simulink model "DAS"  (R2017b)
settings: Solver=FixedStepDiscrete  StartTime=0.0  StopTime=10.0  FixedStep=0.01  RelTol=1e-3  EnableMultiTasking=on
undefined symbols (not defined in the file): CcDAS_ACModeCurtLim_A, CcDAS_ACModeCurtTiLim_ms, CcDAS_BMSOperationConfirmTi_ms, CcDAS_CellMaxTempLim1_C, CcDAS_CellMaxTempLim2_C, CcDAS_CellMaxTempLim3_C, CcDAS_CellMaxTempLim4_C, CcDAS_CellMinTempHiLim_C, CcDAS_CellMinTempLowLim_C, CcDAS_CellMinTempMidLim_C, CcDAS_CellTempDiffLim_C, CcDAS_DCModeCurtTiLim_ms, CcDAS_HVSafetyNVMStoreTi_ms, CcDAS_OCVSOCDiffLim1_numb, CcDAS_OCVSOCDiffLim2_numb, CcDAS_PackCurrLim_A, CcDAS_SOCHighLim_numb, CcDAS_SOCLowerLim_numb, CcDAS_SOHLowerLim_numb, CcDAS_SOHLowerLimSale_numb, DAS_MIN2MS_NUMB, DAS_RUNTIME100_MS, DAS_RUNTIME10_MS, DAS_STATSTIMEMAX_MIN, DAS_STATSTIMEMIN_MIN, DAS_STATSTIMESMAX_NUMB, DAS_STATSTIMESMIN_NUMB, DAS_TIMESONE_NUMB, Enum_CTCCtrCtlConnMode
libraries: AIWAYS_Powertrain_BMS_lib x268
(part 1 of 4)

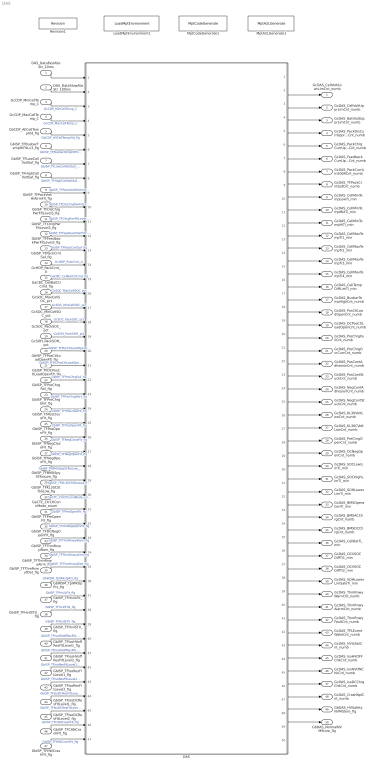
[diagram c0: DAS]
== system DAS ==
  DAS_DataFastAbsStr_10ms : Inport
  DAS_DataSlowAbsStr_100ms : Inport  Port=2
  GcCDP_MinCellTemp_C : Inport  Port=3
  GcCDP_MaxCellTemp_C : Inport  Port=4
  GbCDP_AllCellTempVld_flg : Inport  Port=5
  GbISP_TFBusbarTempHiFltLv3_flg : Inport  Port=6
  GbISP_TFLowCellVoltSaf_flg : Inport  Port=7
  GbISP_TFHighCellVoltSaf_flg : Inport  Port=8
  GbISP_TFPackVoltHiAlrmFlt_flg : Inport  Port=9
  GbISP_TFDisChrgPwrFltLevel3_flg : Inport  Port=10
  GbISP_TFChrgPwrFltLevel3_flg : Inport  Port=11
  GbISP_TFFeedbackPwrFltLevel3_flg : Inport  Port=12
  GbISP_TFPackCrntSaf_flg : Inport  Port=13
  GcHDP_PackCrnt_A : Inport  Port=14
  GaCBC_CellBalCtlCmd_flg : Inport  Port=15
  GcSOC_MaxCellSOC_pct : Inport  Port=16
  GcSOC_MinCellSOC_pct : Inport  Port=17
  GcSOC_PackSOC_pct : Inport  Port=18
  GcSOH_PackSOH_pct : Inport  Port=19
  GbISP_TFPosCtlLoadOpenFlt_flg : Inport  Port=20
  GbISP_TFDCPosCtlLoadOpenFlt_flg : Inport  Port=21
  GbISP_TFPreChrgFail_flg : Inport  Port=22
  GbISP_TFPreChrgShrt_flg : Inport  Port=23
  GbISP_TFPosCloseFlt_flg : Inport  Port=24
  GbISP_TFPosOpenFlt_flg : Inport  Port=25
  GbISP_TFNegCloseFlt_flg : Inport  Port=26
  GbISP_TFNegOpenFlt_flg : Inport  Port=27
  GbISP_TFBMUSpyStTooLow_flg : Inport  Port=28
  GbISP_TFKL30CStTooLow_flg : Inport  Port=29
  GeCTC_CtrCtlConnMode_enum : Inport  Port=30
  GbISP_TFPreOpenFlt_flg : Inport  Port=31
  GbISP_TFDCNegOpenFlt_flg : Inport  Port=32
  GbISP_TFThmRnwyWarn_flg : Inport  Port=33
  GbISP_TFThmRnwyAlrm_flg : Inport  Port=34
  GbISP_TFThmRnwyfDet_flg : Inport  Port=35
  GbWSM_TplWkUpPrs_flg : Inport  Port=36
  GbISP_TFHvilLFlt_flg : Inport  Port=37
  GbISP_TFHvilSTG_flg : Inport  Port=38
  GbISP_TFHvilSTV_flg : Inport  Port=39
  GbISP_TFIsoHVoffResFltLevel1_flg : Inport  Port=40
  GbISP_TFIsoHVoffResFltLevel2_flg : Inport  Port=41
  GbISP_TFIsoResFltLevel1_flg : Inport  Port=42
  GbISP_TFIsoResFltLevel2_flg : Inport  Port=43
  GbISP_TFIsoDCResFltLevel1_flg : Inport  Port=44
  GbISP_TFIsoDCResFltLevel2_flg : Inport  Port=45
  GbISP_TFCANCrashFlt_flg : Inport  Port=46
  GbISP_TFHWCrashFlt_flg : Inport  Port=47
  DAS : Subsystem
  LoadMptEnvironment1 : AIWAYS_Powertrain_BMS_lib/Config/LoadMptEnvironment  ProjectName=Comm  SuppierID=NewPlatformUAES
  MptA2LGenerate1 : AIWAYS_Powertrain_BMS_lib/Config/MptA2LGenerate  SystemSampleTime=-1
  MptCodeGenerate1 : AIWAYS_Powertrain_BMS_lib/Config/MptCodeGenerate  SystemSampleTime=-1
  Revision1 : AIWAYS_Powertrain_BMS_lib/Config/Revision  curVersion='M104C103'  newVersion='M104C103'
  GcDAS_CellVoltLowrLimCnt_numb : Outport
  GcDAS_CellVoltUpprLimCnt_numb : Outport  Port=2
  GcDAS_BattVoltUpprLimCnt_numb : Outport  Port=3
  GcDAS_PackDisCurrUpprLimCnt_numb : Outport  Port=4
  GcDAS_PackChrgCurrUpprLimCnt_numb : Outport  Port=5
  GcDAS_FeedbackCurrUpprLimCnt_numb : Outport  Port=6
  GcDAS_PackCurrLim500ACnt_numb : Outport  Port=7
  GcDAS_TFPackCrntSafCnt_numb : Outport  Port=8
  GcDAS_CellMinTempLowTi_min : Outport  Port=9
  GcDAS_CellMinTempMidTi_min : Outport  Port=10
  GcDAS_CellMinTempHiTi_min : Outport  Port=11
  GcDAS_CellMaxTempTi1_min : Outport  Port=12
  GcDAS_CellMaxTempTi2_min : Outport  Port=13
  GcDAS_CellMaxTempTi3_min : Outport  Port=14
  GcDAS_CellMaxTempTi4_min : Outport  Port=15
  GcDAS_CellTempDiffLimTi_min : Outport  Port=16
  GcDAS_BusbarTempHighCnt_numb : Outport  Port=17
  GcDAS_PosCtlLoadOpenCnt_numb : Outport  Port=18
  GcDAS_DCPosCtlLoadOpenCnt_numb : Outport  Port=19
  GcDAS_PreChrgFailCnt_numb : Outport  Port=20
  GcDAS_PreChrgOvrCurrCnt_numb : Outport  Port=21
  GcDAS_PosContAdhesionCnt_numb : Outport  Port=22
  GcDAS_PosContStuckCnt_numb : Outport  Port=23
  GcDAS_NegContAdhesionCnt_numb : Outport  Port=24
  GcDAS_NegContStuckCnt_numb : Outport  Port=25
  GcDAS_KL30VoltLowCnt_numb : Outport  Port=26
  GcDAS_KL30CVoltLowCnt_numb : Outport  Port=27
  GcDAS_PreChrgOpenCnt_numb : Outport  Port=28
  GcDAS_DCNegOpenCnt_numb : Outport  Port=29
  GcDAS_SOCLowLimTi_min : Outport  Port=30
  GcDAS_SOCHighLimTi_min : Outport  Port=31
  GcDAS_SOHLowerLimTi_min : Outport  Port=32
  GcDAS_BMSOperationTi_min : Outport  Port=33
  GcDAS_BMSACChrgCnt_numb : Outport  Port=34
  GcDAS_BMSDCChrgCnt_numb : Outport  Port=35
  GcDAS_CellBalTi_min : Outport  Port=36
  GcDAS_OCVSOCDiffTi1_min : Outport  Port=37
  GcDAS_OCVSOCDiffTi2_min : Outport  Port=38
  GcDAS_SOHLowerLimSaleTi_min : Outport  Port=39
  GcDAS_ThmRnwyWarnCnt_numb : Outport  Port=40
  GcDAS_ThmRnwyAlarmCnt_numb : Outport  Port=41
  GcDAS_ThmRnwyFaultCnt_numb : Outport  Port=42
  GcDAS_TPLEventWakeCnt_numb : Outport  Port=43
  GcDAS_HVILFailCnt_numb : Outport  Port=44
  GcDAS_IsoHVOFFChkCnt_numb : Outport  Port=45
  GcDAS_IsoHVONChkCnt_numb : Outport  Port=46
  GcDAS_IsoDCChrgChkCnt_numb : Outport  Port=47
  GcDAS_CrashNplCnt_numb : Outport  Port=48
  GbDAS_HVSafetyNVMStore_flg : Outport  Port=49
  GbDAS_NormalNVMStore_flg : Outport  Port=50
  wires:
  DAS_DataFastAbsStr_10ms/1 -> DAS/1(DAS_DataFastAbsStr_10ms)
  DAS_DataSlowAbsStr_100ms/1 -> DAS/2(DAS_DataSlowAbsStr_100ms)
  GcCDP_MinCellTemp_C/1 -> DAS/3(GcCDP_MinCellTemp_C)  "GcCDP_MinCellTemp_C"
  GcCDP_MaxCellTemp_C/1 -> DAS/4(GcCDP_MaxCellTemp_C)  "GcCDP_MaxCellTemp_C"
  GbCDP_AllCellTempVld_flg/1 -> DAS/5(GbCDP_AllCellTempVld_flg)  "GbCDP_AllCellTempVld_flg"
  GbISP_TFBusbarTempHiFltLv3_flg/1 -> DAS/6(GbISP_TFBusbarTempHiFltLv3_flg)  "GbISP_TFBusbarTempHiFltLv3_flg"
  GbISP_TFLowCellVoltSaf_flg/1 -> DAS/7(GbISP_TFLowCellVoltSaf_flg)  "GbISP_TFLowCellVoltSaf_flg"
  GbISP_TFHighCellVoltSaf_flg/1 -> DAS/8(GbISP_TFHighCellVoltSaf_flg)  "GbISP_TFHighCellVoltSaf_flg"
  GbISP_TFPackVoltHiAlrmFlt_flg/1 -> DAS/9(GbISP_TFPackVoltHiAlrmFlt_flg)  "GbISP_TFPackVoltHiAlrmFlt_flg"
  GbISP_TFDisChrgPwrFltLevel3_flg/1 -> DAS/10(GbISP_TFDisChrgPwrFltLevel3_flg)  "GbISP_TFDisChrgPwrFltLevel3_flg"
  GbISP_TFChrgPwrFltLevel3_flg/1 -> DAS/11(GbISP_TFChrgPwrFltLevel3_flg)  "GbISP_TFChrgPwrFltLevel3_flg"
  GbISP_TFFeedbackPwrFltLevel3_flg/1 -> DAS/12(GbISP_TFFeedbackPwrFltLevel3_flg)  "GbISP_TFFeedbackPwrFltLevel3_flg"
  GbISP_TFPackCrntSaf_flg/1 -> DAS/13(GbISP_TFPackCrntSaf_flg)  "GbISP_TFPackCrntSaf_flg"
  GcHDP_PackCrnt_A/1 -> DAS/14(GcHDP_PackCrnt_A)  "GcHDP_PackCrnt_A"
  GaCBC_CellBalCtlCmd_flg/1 -> DAS/15(GaCBC_CellBalCtlCmd_flg)  "GaCBC_CellBalCtlCmd_flg"
  GcSOC_MaxCellSOC_pct/1 -> DAS/16(GcSOC_MaxCellSOC_pct)  "GcSOC_MaxCellSOC_pct"
  GcSOC_MinCellSOC_pct/1 -> DAS/17(GcSOC_MinCellSOC_pct)  "GcSOC_MinCellSOC_pct"
  GcSOC_PackSOC_pct/1 -> DAS/18(GcSOC_PackSOC_pct)  "GcSOC_PackSOC_pct"
  GcSOH_PackSOH_pct/1 -> DAS/19(GcSOH_PackSOH_pct)  "GcSOH_PackSOH_pct"
  GbISP_TFPreChrgFail_flg/1 -> DAS/22(GbISP_TFPreChrgFail_flg)  "GbISP_TFPreChrgFail_flg"
  GbISP_TFPosCloseFlt_flg/1 -> DAS/24(GbISP_TFPosCloseFlt_flg)  "GbISP_TFPosCloseFlt_flg"
  GbISP_TFPosOpenFlt_flg/1 -> DAS/25(GbISP_TFPosOpenFlt_flg)  "GbISP_TFPosOpenFlt_flg"
  GbISP_TFNegCloseFlt_flg/1 -> DAS/26(GbISP_TFNegCloseFlt_flg)  "GbISP_TFNegCloseFlt_flg"
  GbISP_TFNegOpenFlt_flg/1 -> DAS/27(GbISP_TFNegOpenFlt_flg)  "GbISP_TFNegOpenFlt_flg"
  GbISP_TFBMUSpyStTooLow_flg/1 -> DAS/28(GbISP_TFBMUSpyStTooLow_flg)  "GbISP_TFBMUSpyStTooLow_flg"
  GbISP_TFKL30CStTooLow_flg/1 -> DAS/29(GbISP_TFKL30CStTooLow_flg)  "GbISP_TFKL30CStTooLow_flg"
  GbISP_TFDCNegOpenFlt_flg/1 -> DAS/32(GbISP_TFDCNegOpenFlt_flg)  "GbISP_TFDCNegOpenFlt_flg"
  GbISP_TFPreOpenFlt_flg/1 -> DAS/31(GbISP_TFPreOpenFlt_flg)  "GbISP_TFPreOpenFlt_flg"
  GeCTC_CtrCtlConnMode_enum/1 -> DAS/30(GeCTC_CtrCtlConnMode_enum)  "GeCTC_CtrCtlConnMode_enum"
  GbISP_TFThmRnwyWarn_flg/1 -> DAS/33(GbISP_TFThmRnwyWarn_flg)  "GbISP_TFThmRnwyWarn_flg"
  GbISP_TFThmRnwyAlrm_flg/1 -> DAS/34(GbISP_TFThmRnwyAlrm_flg)  "GbISP_TFThmRnwyAlrm_flg"
  GbISP_TFThmRnwyfDet_flg/1 -> DAS/35(GbISP_TFThmRnwyfDet_flg)  "GbISP_TFThmRnwyfDet_flg"
  GbWSM_TplWkUpPrs_flg/1 -> DAS/36(GbWSM_TplWkUpPrs_flg)  "GbWSM_TplWkUpPrs_flg"
  GbISP_TFHvilLFlt_flg/1 -> DAS/37(GbISP_TFHvilLFlt_flg)  "GbISP_TFHvilLFlt_flg"
  GbISP_TFHvilSTG_flg/1 -> DAS/38(GbISP_TFHvilSTG_flg)  "GbISP_TFHvilSTG_flg"
  GbISP_TFHvilSTV_flg/1 -> DAS/39(GbISP_TFHvilSTV_flg)  "GbISP_TFHvilSTV_flg"
  GbISP_TFIsoHVoffResFltLevel1_flg/1 -> DAS/40(GbISP_TFIsoHVoffResFltLevel1_flg)  "GbISP_TFIsoHVoffResFltLevel1_flg"
  GbISP_TFIsoHVoffResFltLevel2_flg/1 -> DAS/41(GbISP_TFIsoHVoffResFltLevel2_flg)  "GbISP_TFIsoHVoffResFltLevel2_flg"
  GbISP_TFIsoResFltLevel1_flg/1 -> DAS/42(GbISP_TFIsoResFltLevel1_flg)  "GbISP_TFIsoResFltLevel1_flg"
  GbISP_TFHWCrashFlt_flg/1 -> DAS/47(GbISP_TFHWCrashFlt_flg)  "GbISP_TFHWCrashFlt_flg"
  GbISP_TFCANCrashFlt_flg/1 -> DAS/46(GbISP_TFCANCrashFlt_flg)  "GbISP_TFCANCrashFlt_flg"
  GbISP_TFIsoDCResFltLevel2_flg/1 -> DAS/45(GbISP_TFIsoDCResFltLevel2_flg)  "GbISP_TFIsoDCResFltLevel2_flg"
  GbISP_TFIsoDCResFltLevel1_flg/1 -> DAS/44(GbISP_TFIsoDCResFltLevel1_flg)  "GbISP_TFIsoDCResFltLevel1_flg"
  GbISP_TFIsoResFltLevel2_flg/1 -> DAS/43(GbISP_TFIsoResFltLevel2_flg)  "GbISP_TFIsoResFltLevel2_flg"
  DAS/1(GcDAS_CellVoltLowrLimCnt_numb) -> GcDAS_CellVoltLowrLimCnt_numb/1
  DAS/2(GcDAS_CellVoltUpprLimCnt_numb) -> GcDAS_CellVoltUpprLimCnt_numb/1
  DAS/3(GcDAS_BattVoltUpprLimCnt_numb) -> GcDAS_BattVoltUpprLimCnt_numb/1
  DAS/4(GcDAS_PackDisCurrUpprLimCnt_numb) -> GcDAS_PackDisCurrUpprLimCnt_numb/1
  DAS/5(GcDAS_PackChrgCurrUpprLimCnt_numb) -> GcDAS_PackChrgCurrUpprLimCnt_numb/1
  DAS/6(GcDAS_FeedbackCurrUpprLimCnt_numb) -> GcDAS_FeedbackCurrUpprLimCnt_numb/1
  DAS/7(GcDAS_PackCurrLim500ACnt_numb) -> GcDAS_PackCurrLim500ACnt_numb/1
  DAS/8(GcDAS_TFPackCrntSafCnt_numb) -> GcDAS_TFPackCrntSafCnt_numb/1
  DAS/9(GcDAS_CellMinTempLowTi_min) -> GcDAS_CellMinTempLowTi_min/1
  DAS/10(GcDAS_CellMinTempMidTi_min) -> GcDAS_CellMinTempMidTi_min/1
  DAS/11(GcDAS_CellMinTempHiTi_min) -> GcDAS_CellMinTempHiTi_min/1
  DAS/12(GcDAS_CellMaxTempTi1_min) -> GcDAS_CellMaxTempTi1_min/1
  DAS/13(GcDAS_CellMaxTempTi2_min) -> GcDAS_CellMaxTempTi2_min/1
  DAS/14(GcDAS_CellMaxTempTi3_min) -> GcDAS_CellMaxTempTi3_min/1
  DAS/15(GcDAS_CellMaxTempTi4_min) -> GcDAS_CellMaxTempTi4_min/1
  DAS/16(GcDAS_CellTempDiffLimTi_min) -> GcDAS_CellTempDiffLimTi_min/1
  DAS/17(GcDAS_BusbarTempHighCnt_numb) -> GcDAS_BusbarTempHighCnt_numb/1
  DAS/18(GcDAS_PosCtlLoadOpenCnt_numb) -> GcDAS_PosCtlLoadOpenCnt_numb/1
  DAS/19(GcDAS_DCPosCtlLoadOpenCnt_numb) -> GcDAS_DCPosCtlLoadOpenCnt_numb/1
  DAS/20(GcDAS_PreChrgFailCnt_numb) -> GcDAS_PreChrgFailCnt_numb/1
  DAS/21(GcDAS_PreChrgOvrCurrCnt_numb) -> GcDAS_PreChrgOvrCurrCnt_numb/1
  DAS/22(GcDAS_PosContAdhesionCnt_numb) -> GcDAS_PosContAdhesionCnt_numb/1
  DAS/23(GcDAS_PosContStuckCnt_numb) -> GcDAS_PosContStuckCnt_numb/1
  DAS/24(GcDAS_NegContAdhesionCnt_numb) -> GcDAS_NegContAdhesionCnt_numb/1
  DAS/25(GcDAS_NegContStuckCnt_numb) -> GcDAS_NegContStuckCnt_numb/1
  DAS/26(GcDAS_KL30VoltLowCnt_numb) -> GcDAS_KL30VoltLowCnt_numb/1
  DAS/27(GcDAS_KL30CVoltLowCnt_numb) -> GcDAS_KL30CVoltLowCnt_numb/1
  DAS/28(GcDAS_PreChrgOpenCnt_numb) -> GcDAS_PreChrgOpenCnt_numb/1
  DAS/29(GcDAS_DCNegOpenCnt_numb) -> GcDAS_DCNegOpenCnt_numb/1
  DAS/30(GcDAS_SOCLowLimTi_min) -> GcDAS_SOCLowLimTi_min/1
  DAS/31(GcDAS_SOCHighLimTi_min) -> GcDAS_SOCHighLimTi_min/1
  DAS/32(GcDAS_SOHLowerLimTi_min) -> GcDAS_SOHLowerLimTi_min/1
  DAS/33(GcDAS_BMSOperationTi_min) -> GcDAS_BMSOperationTi_min/1
  DAS/34(GcDAS_BMSACChrgCnt_numb) -> GcDAS_BMSACChrgCnt_numb/1
  DAS/35(GcDAS_BMSDCChrgCnt_numb) -> GcDAS_BMSDCChrgCnt_numb/1
  DAS/36(GcDAS_CellBalTi_min) -> GcDAS_CellBalTi_min/1
  DAS/37(GcDAS_OCVSOCDiffTi1_min) -> GcDAS_OCVSOCDiffTi1_min/1
  DAS/38(GcDAS_OCVSOCDiffTi2_min) -> GcDAS_OCVSOCDiffTi2_min/1
  DAS/39(GcDAS_SOHLowerLimSaleTi_min) -> GcDAS_SOHLowerLimSaleTi_min/1
  DAS/40(GcDAS_ThmRnwyWarnCnt_numb) -> GcDAS_ThmRnwyWarnCnt_numb/1
  DAS/41(GcDAS_ThmRnwyAlarmCnt_numb) -> GcDAS_ThmRnwyAlarmCnt_numb/1
  DAS/42(GcDAS_ThmRnwyFaultCnt_numb) -> GcDAS_ThmRnwyFaultCnt_numb/1
  DAS/43(GcDAS_TPLEventWakeCnt_numb) -> GcDAS_TPLEventWakeCnt_numb/1
  DAS/44(GcDAS_HVILFailCnt_numb) -> GcDAS_HVILFailCnt_numb/1
  DAS/45(GcDAS_IsoHVOFFChkCnt_numb) -> GcDAS_IsoHVOFFChkCnt_numb/1
  DAS/46(GcDAS_IsoHVONChkCnt_numb) -> GcDAS_IsoHVONChkCnt_numb/1
  DAS/47(GcDAS_IsoDCChrgChkCnt_numb) -> GcDAS_IsoDCChrgChkCnt_numb/1
  DAS/48(GcDAS_CrashNplCnt_numb) -> GcDAS_CrashNplCnt_numb/1
  GbISP_TFPosCtlLoadOpenFlt_flg/1 -> DAS/20(GbISP_TFPosCtlLoadOpenFlt_flg)  "GbISP_TFPosCtlLoadOpenFlt_flg"
  GbISP_TFDCPosCtlLoadOpenFlt_flg/1 -> DAS/21(GbISP_TFDCPosCtlLoadOpenFlt_flg)  "GbISP_TFDCPosCtlLoadOpenFlt_flg"
  GbISP_TFPreChrgShrt_flg/1 -> DAS/23(GbISP_TFPreChrgShrt_flg)  "GbISP_TFPreChrgShrt_flg"
  DAS/49(GbDAS_HVSafetyNVMStore_flg) -> GbDAS_HVSafetyNVMStore_flg/1
  DAS/50(GbDAS_NormalNVMStore_flg) -> GbDAS_NormalNVMStore_flg/1

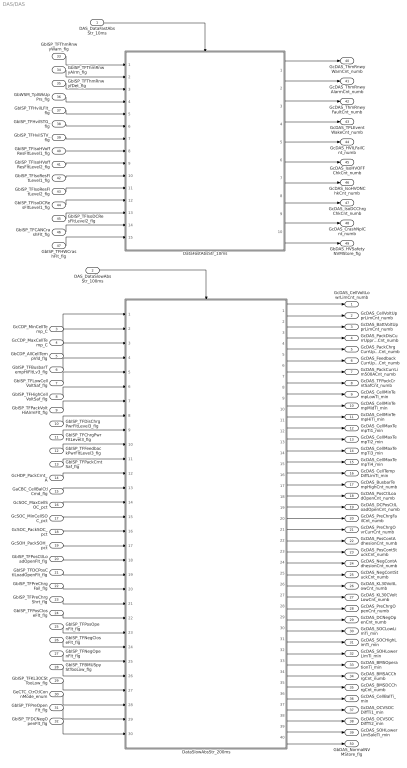
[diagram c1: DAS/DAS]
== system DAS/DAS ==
  DAS_DataFastAbsStr_10ms : Inport
  DAS_DataSlowAbsStr_100ms : Inport  Port=2
  GcCDP_MinCellTemp_C : Inport  Port=3
  GcCDP_MaxCellTemp_C : Inport  Port=4
  GbCDP_AllCellTempVld_flg : Inport  Port=5
  GbISP_TFBusbarTempHiFltLv3_flg : Inport  Port=6
  GbISP_TFLowCellVoltSaf_flg : Inport  Port=7
  GbISP_TFHighCellVoltSaf_flg : Inport  Port=8
  GbISP_TFPackVoltHiAlrmFlt_flg : Inport  Port=9
  GbISP_TFDisChrgPwrFltLevel3_flg : Inport  Port=10
  GbISP_TFChrgPwrFltLevel3_flg : Inport  Port=11
  GbISP_TFFeedbackPwrFltLevel3_flg : Inport  Port=12
  GbISP_TFPackCrntSaf_flg : Inport  Port=13
  GcHDP_PackCrnt_A : Inport  Port=14
  GaCBC_CellBalCtlCmd_flg : Inport  Port=15
  GcSOC_MaxCellSOC_pct : Inport  Port=16
  GcSOC_MinCellSOC_pct : Inport  Port=17
  GcSOC_PackSOC_pct : Inport  Port=18
  GcSOH_PackSOH_pct : Inport  Port=19
  GbISP_TFPosCtlLoadOpenFlt_flg : Inport  Port=20
  GbISP_TFDCPosCtlLoadOpenFlt_flg : Inport  Port=21
  GbISP_TFPreChrgFail_flg : Inport  Port=22
  GbISP_TFPreChrgShrt_flg : Inport  Port=23
  GbISP_TFPosCloseFlt_flg : Inport  Port=24
  GbISP_TFPosOpenFlt_flg : Inport  Port=25
  GbISP_TFNegCloseFlt_flg : Inport  Port=26
  GbISP_TFNegOpenFlt_flg : Inport  Port=27
  GbISP_TFBMUSpyStTooLow_flg : Inport  Port=28
  GbISP_TFKL30CStTooLow_flg : Inport  Port=29
  GeCTC_CtrCtlConnMode_enum : Inport  Port=30
  GbISP_TFPreOpenFlt_flg : Inport  Port=31
  GbISP_TFDCNegOpenFlt_flg : Inport  Port=32
  GbISP_TFThmRnwyWarn_flg : Inport  Port=33
  GbISP_TFThmRnwyAlrm_flg : Inport  Port=34
  GbISP_TFThmRnwyfDet_flg : Inport  Port=35
  GbWSM_TplWkUpPrs_flg : Inport  Port=36
  GbISP_TFHvilLFlt_flg : Inport  Port=37
  GbISP_TFHvilSTG_flg : Inport  Port=38
  GbISP_TFHvilSTV_flg : Inport  Port=39
  GbISP_TFIsoHVoffResFltLevel1_flg : Inport  Port=40
  GbISP_TFIsoHVoffResFltLevel2_flg : Inport  Port=41
  GbISP_TFIsoResFltLevel1_flg : Inport  Port=42
  GbISP_TFIsoResFltLevel2_flg : Inport  Port=43
  GbISP_TFIsoDCResFltLevel1_flg : Inport  Port=44
  GbISP_TFIsoDCResFltLevel2_flg : Inport  Port=45
  GbISP_TFCANCrashFlt_flg : Inport  Port=46
  GbISP_TFHWCrashFlt_flg : Inport  Port=47
  DataFastAbsStr_10ms : Subsystem
  DataSlowAbsStr_200ms : Subsystem
  GcDAS_CellVoltLowrLimCnt_numb : Outport
  GcDAS_CellVoltUpprLimCnt_numb : Outport  Port=2
  GcDAS_BattVoltUpprLimCnt_numb : Outport  Port=3
  GcDAS_PackDisCurrUpprLimCnt_numb : Outport  Port=4
  GcDAS_PackChrgCurrUpprLimCnt_numb : Outport  Port=5
  GcDAS_FeedbackCurrUpprLimCnt_numb : Outport  Port=6
  GcDAS_PackCurrLim500ACnt_numb : Outport  Port=7
  GcDAS_TFPackCrntSafCnt_numb : Outport  Port=8
  GcDAS_CellMinTempLowTi_min : Outport  Port=9
  GcDAS_CellMinTempMidTi_min : Outport  Port=10
  GcDAS_CellMinTempHiTi_min : Outport  Port=11
  GcDAS_CellMaxTempTi1_min : Outport  Port=12
  GcDAS_CellMaxTempTi2_min : Outport  Port=13
  GcDAS_CellMaxTempTi3_min : Outport  Port=14
  GcDAS_CellMaxTempTi4_min : Outport  Port=15
  GcDAS_CellTempDiffLimTi_min : Outport  Port=16
  GcDAS_BusbarTempHighCnt_numb : Outport  Port=17
  GcDAS_PosCtlLoadOpenCnt_numb : Outport  Port=18
  GcDAS_DCPosCtlLoadOpenCnt_numb : Outport  Port=19
  GcDAS_PreChrgFailCnt_numb : Outport  Port=20
  GcDAS_PreChrgOvrCurrCnt_numb : Outport  Port=21
  GcDAS_PosContAdhesionCnt_numb : Outport  Port=22
  GcDAS_PosContStuckCnt_numb : Outport  Port=23
  GcDAS_NegContAdhesionCnt_numb : Outport  Port=24
  GcDAS_NegContStuckCnt_numb : Outport  Port=25
  GcDAS_KL30VoltLowCnt_numb : Outport  Port=26
  GcDAS_KL30CVoltLowCnt_numb : Outport  Port=27
  GcDAS_PreChrgOpenCnt_numb : Outport  Port=28
  GcDAS_DCNegOpenCnt_numb : Outport  Port=29
  GcDAS_SOCLowLimTi_min : Outport  Port=30
  GcDAS_SOCHighLimTi_min : Outport  Port=31
  GcDAS_SOHLowerLimTi_min : Outport  Port=32
  GcDAS_BMSOperationTi_min : Outport  Port=33
  GcDAS_BMSACChrgCnt_numb : Outport  Port=34
  GcDAS_BMSDCChrgCnt_numb : Outport  Port=35
  GcDAS_CellBalTi_min : Outport  Port=36
  GcDAS_OCVSOCDiffTi1_min : Outport  Port=37
  GcDAS_OCVSOCDiffTi2_min : Outport  Port=38
  GcDAS_SOHLowerLimSaleTi_min : Outport  Port=39
  GcDAS_ThmRnwyWarnCnt_numb : Outport  Port=40
  GcDAS_ThmRnwyAlarmCnt_numb : Outport  Port=41
  GcDAS_ThmRnwyFaultCnt_numb : Outport  Port=42
  GcDAS_TPLEventWakeCnt_numb : Outport  Port=43
  GcDAS_HVILFailCnt_numb : Outport  Port=44
  GcDAS_IsoHVOFFChkCnt_numb : Outport  Port=45
  GcDAS_IsoHVONChkCnt_numb : Outport  Port=46
  GcDAS_IsoDCChrgChkCnt_numb : Outport  Port=47
  GcDAS_CrashNplCnt_numb : Outport  Port=48
  GbDAS_HVSafetyNVMStore_flg : Outport  Port=49
  GbDAS_NormalNVMStore_flg : Outport  Port=50
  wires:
  DAS_DataSlowAbsStr_100ms/1 -> DataSlowAbsStr_200ms/Trigger
  DAS_DataFastAbsStr_10ms/1 -> DataFastAbsStr_10ms/Trigger
  GcCDP_MinCellTemp_C/1 -> DataSlowAbsStr_200ms/1(GcCDP_MinCellTemp_C)
  GcCDP_MaxCellTemp_C/1 -> DataSlowAbsStr_200ms/2(GcCDP_MaxCellTemp_C)
  GbCDP_AllCellTempVld_flg/1 -> DataSlowAbsStr_200ms/3(GbCDP_AllCellTempVld_flg)
  GbISP_TFBusbarTempHiFltLv3_flg/1 -> DataSlowAbsStr_200ms/4(GbISP_TFBusbarTempHiFltLv3_flg)
  GbISP_TFLowCellVoltSaf_flg/1 -> DataSlowAbsStr_200ms/5(GbISP_TFLowCellVoltSaf_flg)
  GbISP_TFHighCellVoltSaf_flg/1 -> DataSlowAbsStr_200ms/6(GbISP_TFHighCellVoltSaf_flg)
  GbISP_TFPackVoltHiAlrmFlt_flg/1 -> DataSlowAbsStr_200ms/7(GbISP_TFPackVoltHiAlrmFlt_flg)
  GbISP_TFDisChrgPwrFltLevel3_flg/1 -> DataSlowAbsStr_200ms/8(GbISP_TFDisChrgPwrFltLevel3_flg)
  GbISP_TFChrgPwrFltLevel3_flg/1 -> DataSlowAbsStr_200ms/9(GbISP_TFChrgPwrFltLevel3_flg)
  GbISP_TFFeedbackPwrFltLevel3_flg/1 -> DataSlowAbsStr_200ms/10(GbISP_TFFeedbackPwrFltLevel3_flg)
  GbISP_TFPackCrntSaf_flg/1 -> DataSlowAbsStr_200ms/11(GbISP_TFPackCrntSaf_flg)
  GcHDP_PackCrnt_A/1 -> DataSlowAbsStr_200ms/12(GcHDP_PackCrnt_A)
  GaCBC_CellBalCtlCmd_flg/1 -> DataSlowAbsStr_200ms/13(GaCBC_CellBalCtlCmd_flg)
  GcSOC_MaxCellSOC_pct/1 -> DataSlowAbsStr_200ms/14(GcSOC_MaxCellSOC_pct)
  GcSOC_MinCellSOC_pct/1 -> DataSlowAbsStr_200ms/15(GcSOC_MinCellSOC_pct)
  GcSOC_PackSOC_pct/1 -> DataSlowAbsStr_200ms/16(GcSOC_PackSOC_pct)
  GcSOH_PackSOH_pct/1 -> DataSlowAbsStr_200ms/17(GcSOH_PackSOH_pct)
  GbISP_TFPosCtlLoadOpenFlt_flg/1 -> DataSlowAbsStr_200ms/18(GbISP_TFPosCtlLoadOpenFlt_flg)
  GbISP_TFDCPosCtlLoadOpenFlt_flg/1 -> DataSlowAbsStr_200ms/19(GbISP_TFDCPosCtlLoadOpenFlt_flg)
  GbISP_TFPreChrgFail_flg/1 -> DataSlowAbsStr_200ms/20(GbISP_TFPreChrgFail_flg)
  GbISP_TFPreChrgShrt_flg/1 -> DataSlowAbsStr_200ms/21(GbISP_TFPreChrgShrt_flg)
  GbISP_TFPosCloseFlt_flg/1 -> DataSlowAbsStr_200ms/22(GbISP_TFPosCloseFlt_flg)
  GbISP_TFPosOpenFlt_flg/1 -> DataSlowAbsStr_200ms/23(GbISP_TFPosOpenFlt_flg)
  GbISP_TFNegCloseFlt_flg/1 -> DataSlowAbsStr_200ms/24(GbISP_TFNegCloseFlt_flg)
  GbISP_TFNegOpenFlt_flg/1 -> DataSlowAbsStr_200ms/25(GbISP_TFNegOpenFlt_flg)
  GbISP_TFBMUSpyStTooLow_flg/1 -> DataSlowAbsStr_200ms/26(GbISP_TFBMUSpyStTooLow_flg)
  GbISP_TFKL30CStTooLow_flg/1 -> DataSlowAbsStr_200ms/27(GbISP_TFKL30CStTooLow_flg)
  GeCTC_CtrCtlConnMode_enum/1 -> DataSlowAbsStr_200ms/28(GeCTC_CtrCtlConnMode_enum)
  GbISP_TFPreOpenFlt_flg/1 -> DataSlowAbsStr_200ms/29(GbISP_TFPreOpenFlt_flg)
  GbISP_TFDCNegOpenFlt_flg/1 -> DataSlowAbsStr_200ms/30(GbISP_TFDCNegOpenFlt_flg)
  DataSlowAbsStr_200ms/1(GcDAS_CellVoltLowrLimCnt_numb) -> GcDAS_CellVoltLowrLimCnt_numb/1
  DataSlowAbsStr_200ms/2(GcDAS_CellVoltUpprLimCnt_numb) -> GcDAS_CellVoltUpprLimCnt_numb/1
  DataSlowAbsStr_200ms/3(GcDAS_BattVoltUpprLimCnt_numb) -> GcDAS_BattVoltUpprLimCnt_numb/1
  DataSlowAbsStr_200ms/4(GcDAS_PackDisCurrUpprLimCnt_numb) -> GcDAS_PackDisCurrUpprLimCnt_numb/1
  DataSlowAbsStr_200ms/5(GcDAS_PackChrgCurrUpprLimCnt_numb) -> GcDAS_PackChrgCurrUpprLimCnt_numb/1
  DataSlowAbsStr_200ms/6(GcDAS_FeedbackCurrUpprLimCnt_numb) -> GcDAS_FeedbackCurrUpprLimCnt_numb/1
  DataSlowAbsStr_200ms/7(GcDAS_PackCurrLim500ACnt_numb) -> GcDAS_PackCurrLim500ACnt_numb/1
  DataSlowAbsStr_200ms/8(GcDAS_TFPackCrntSafCnt_numb) -> GcDAS_TFPackCrntSafCnt_numb/1
  DataSlowAbsStr_200ms/9(GcDAS_CellMinTempLowTi_min) -> GcDAS_CellMinTempLowTi_min/1
  DataSlowAbsStr_200ms/10(GcDAS_CellMinTempMidTi_min) -> GcDAS_CellMinTempMidTi_min/1
  DataSlowAbsStr_200ms/11(GcDAS_CellMinTempHiTi_min) -> GcDAS_CellMinTempHiTi_min/1
  DataSlowAbsStr_200ms/12(GcDAS_CellMaxTempTi1_min) -> GcDAS_CellMaxTempTi1_min/1
  DataSlowAbsStr_200ms/13(GcDAS_CellMaxTempTi2_min) -> GcDAS_CellMaxTempTi2_min/1
  DataSlowAbsStr_200ms/14(GcDAS_CellMaxTempTi3_min) -> GcDAS_CellMaxTempTi3_min/1
  DataSlowAbsStr_200ms/15(GcDAS_CellMaxTempTi4_min) -> GcDAS_CellMaxTempTi4_min/1
  DataSlowAbsStr_200ms/16(GcDAS_CellTempDiffLimTi_min) -> GcDAS_CellTempDiffLimTi_min/1
  DataSlowAbsStr_200ms/17(GcDAS_BusbarTempHighCnt_numb) -> GcDAS_BusbarTempHighCnt_numb/1
  DataSlowAbsStr_200ms/24(GcDAS_NegContAdhesionCnt_numb) -> GcDAS_NegContAdhesionCnt_numb/1
  DataSlowAbsStr_200ms/28(GcDAS_PreChrgOpenCnt_numb) -> GcDAS_PreChrgOpenCnt_numb/1
  DataSlowAbsStr_200ms/19(GcDAS_DCPosCtlLoadOpenCnt_numb) -> GcDAS_DCPosCtlLoadOpenCnt_numb/1
  DataSlowAbsStr_200ms/20(GcDAS_PreChrgFailCnt_numb) -> GcDAS_PreChrgFailCnt_numb/1
  DataSlowAbsStr_200ms/21(GcDAS_PreChrgOvrCurrCnt_numb) -> GcDAS_PreChrgOvrCurrCnt_numb/1
  DataSlowAbsStr_200ms/29(GcDAS_DCNegOpenCnt_numb) -> GcDAS_DCNegOpenCnt_numb/1
  DataSlowAbsStr_200ms/18(GcDAS_PosCtlLoadOpenCnt_numb) -> GcDAS_PosCtlLoadOpenCnt_numb/1
  DataSlowAbsStr_200ms/27(GcDAS_KL30CVoltLowCnt_numb) -> GcDAS_KL30CVoltLowCnt_numb/1
  DataSlowAbsStr_200ms/23(GcDAS_PosContStuckCnt_numb) -> GcDAS_PosContStuckCnt_numb/1
  DataSlowAbsStr_200ms/22(GcDAS_PosContAdhesionCnt_numb) -> GcDAS_PosContAdhesionCnt_numb/1
  DataSlowAbsStr_200ms/26(GcDAS_KL30VoltLowCnt_numb) -> GcDAS_KL30VoltLowCnt_numb/1
  DataSlowAbsStr_200ms/25(GcDAS_NegContStuckCnt_numb) -> GcDAS_NegContStuckCnt_numb/1
  DataSlowAbsStr_200ms/30(GcDAS_SOCLowLimTi_min) -> GcDAS_SOCLowLimTi_min/1
  DataSlowAbsStr_200ms/31(GcDAS_SOCHighLimTi_min) -> GcDAS_SOCHighLimTi_min/1
  DataSlowAbsStr_200ms/32(GcDAS_SOHLowerLimTi_min) -> GcDAS_SOHLowerLimTi_min/1
  DataSlowAbsStr_200ms/33(GcDAS_BMSOperationTi_min) -> GcDAS_BMSOperationTi_min/1
  DataSlowAbsStr_200ms/34(GcDAS_BMSACChrgCnt_numb) -> GcDAS_BMSACChrgCnt_numb/1
  DataSlowAbsStr_200ms/35(GcDAS_BMSDCChrgCnt_numb) -> GcDAS_BMSDCChrgCnt_numb/1
  DataSlowAbsStr_200ms/36(GcDAS_CellBalTi_min) -> GcDAS_CellBalTi_min/1
  DataSlowAbsStr_200ms/37(GcDAS_OCVSOCDiffTi1_min) -> GcDAS_OCVSOCDiffTi1_min/1
  DataSlowAbsStr_200ms/38(GcDAS_OCVSOCDiffTi2_min) -> GcDAS_OCVSOCDiffTi2_min/1
  DataSlowAbsStr_200ms/39(GcDAS_SOHLowerLimSaleTi_min) -> GcDAS_SOHLowerLimSaleTi_min/1
  GbISP_TFThmRnwyWarn_flg/1 -> DataFastAbsStr_10ms/1(GbISP_TFThmRnwyWarn_flg)
  GbISP_TFThmRnwyAlrm_flg/1 -> DataFastAbsStr_10ms/2(GbISP_TFThmRnwyAlrm_flg)
  GbISP_TFThmRnwyfDet_flg/1 -> DataFastAbsStr_10ms/3(GbISP_TFThmRnwyfDet_flg)
  GbWSM_TplWkUpPrs_flg/1 -> DataFastAbsStr_10ms/4(GbWSM_TplWkUpPrs_flg)
  GbISP_TFHvilLFlt_flg/1 -> DataFastAbsStr_10ms/5(GbISP_TFHvilLFlt_flg)
  GbISP_TFHvilSTG_flg/1 -> DataFastAbsStr_10ms/6(GbISP_TFHvilSTG_flg)
  GbISP_TFHvilSTV_flg/1 -> DataFastAbsStr_10ms/7(GbISP_TFHvilSTV_flg)
  GbISP_TFIsoHVoffResFltLevel1_flg/1 -> DataFastAbsStr_10ms/8(GbISP_TFIsoHVoffResFltLevel1_flg)
  GbISP_TFIsoHVoffResFltLevel2_flg/1 -> DataFastAbsStr_10ms/9(GbISP_TFIsoHVoffResFltLevel2_flg)
  GbISP_TFIsoResFltLevel1_flg/1 -> DataFastAbsStr_10ms/10(GbISP_TFIsoResFltLevel1_flg)
  GbISP_TFIsoResFltLevel2_flg/1 -> DataFastAbsStr_10ms/11(GbISP_TFIsoResFltLevel2_flg)
  GbISP_TFIsoDCResFltLevel1_flg/1 -> DataFastAbsStr_10ms/12(GbISP_TFIsoDCResFltLevel1_flg)
  GbISP_TFIsoDCResFltLevel2_flg/1 -> DataFastAbsStr_10ms/13(GbISP_TFIsoDCResFltLevel2_flg)
  GbISP_TFCANCrashFlt_flg/1 -> DataFastAbsStr_10ms/14(GbISP_TFCANCrashFlt_flg)
  GbISP_TFHWCrashFlt_flg/1 -> DataFastAbsStr_10ms/15(GbISP_TFHWCrashFlt_flg)
  DataFastAbsStr_10ms/1(GcDAS_ThmRnwyWarnCnt_numb) -> GcDAS_ThmRnwyWarnCnt_numb/1
  DataFastAbsStr_10ms/2(GcDAS_ThmRnwyAlarmCnt_numb) -> GcDAS_ThmRnwyAlarmCnt_numb/1
  DataFastAbsStr_10ms/3(GcDAS_ThmRnwyFaultCnt_numb) -> GcDAS_ThmRnwyFaultCnt_numb/1
  DataFastAbsStr_10ms/4(GcDAS_TPLEventWakeCnt_numb) -> GcDAS_TPLEventWakeCnt_numb/1
  DataFastAbsStr_10ms/5(GcDAS_HVILFailCnt_numb) -> GcDAS_HVILFailCnt_numb/1
  DataFastAbsStr_10ms/6(GcDAS_IsoHVOFFChkCnt_numb) -> GcDAS_IsoHVOFFChkCnt_numb/1
  DataFastAbsStr_10ms/7(GcDAS_IsoHVONChkCnt_numb) -> GcDAS_IsoHVONChkCnt_numb/1
  DataFastAbsStr_10ms/8(GcDAS_IsoDCChrgChkCnt_numb) -> GcDAS_IsoDCChrgChkCnt_numb/1
  DataFastAbsStr_10ms/9(GcDAS_CrashNplCnt_numb) -> GcDAS_CrashNplCnt_numb/1
  DataFastAbsStr_10ms/10(GbDAS_HVSafetyNVMStore_flg) -> GbDAS_HVSafetyNVMStore_flg/1
  DataSlowAbsStr_200ms/40(GbDAS_NormalNVMStore_flg) -> GbDAS_NormalNVMStore_flg/1

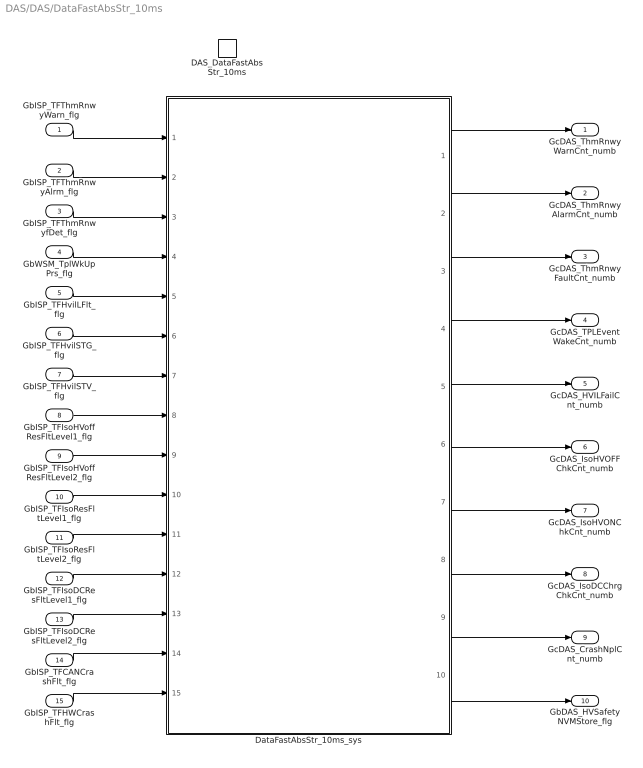
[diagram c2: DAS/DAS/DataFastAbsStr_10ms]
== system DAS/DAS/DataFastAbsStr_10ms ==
  GbISP_TFThmRnwyWarn_flg : Inport
  GbISP_TFThmRnwyAlrm_flg : Inport  Port=2
  GbISP_TFThmRnwyfDet_flg : Inport  Port=3
  GbWSM_TplWkUpPrs_flg : Inport  Port=4
  GbISP_TFHvilLFlt_flg : Inport  Port=5
  GbISP_TFHvilSTG_flg : Inport  Port=6
  GbISP_TFHvilSTV_flg : Inport  Port=7
  GbISP_TFIsoHVoffResFltLevel1_flg : Inport  Port=8
  GbISP_TFIsoHVoffResFltLevel2_flg : Inport  Port=9
  GbISP_TFIsoResFltLevel1_flg : Inport  Port=10
  GbISP_TFIsoResFltLevel2_flg : Inport  Port=11
  GbISP_TFIsoDCResFltLevel1_flg : Inport  Port=12
  GbISP_TFIsoDCResFltLevel2_flg : Inport  Port=13
  GbISP_TFCANCrashFlt_flg : Inport  Port=14
  GbISP_TFHWCrashFlt_flg : Inport  Port=15
  DAS_DataFastAbsStr_10ms : TriggerPort  TriggerType=function-call  VariantControl=(inherit)
  DataFastAbsStr_10ms_sys : Subsystem
  GcDAS_ThmRnwyWarnCnt_numb : Outport
  GcDAS_ThmRnwyAlarmCnt_numb : Outport  Port=2
  GcDAS_ThmRnwyFaultCnt_numb : Outport  Port=3
  GcDAS_TPLEventWakeCnt_numb : Outport  Port=4
  GcDAS_HVILFailCnt_numb : Outport  Port=5
  GcDAS_IsoHVOFFChkCnt_numb : Outport  Port=6
  GcDAS_IsoHVONChkCnt_numb : Outport  Port=7
  GcDAS_IsoDCChrgChkCnt_numb : Outport  Port=8
  GcDAS_CrashNplCnt_numb : Outport  Port=9
  GbDAS_HVSafetyNVMStore_flg : Outport  Port=10
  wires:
  GbISP_TFThmRnwyWarn_flg/1 -> DataFastAbsStr_10ms_sys/1(GbISP_TFThmRnwyWarn_flg)
  GbISP_TFThmRnwyAlrm_flg/1 -> DataFastAbsStr_10ms_sys/2(GbISP_TFThmRnwyAlrm_flg)
  GbISP_TFThmRnwyfDet_flg/1 -> DataFastAbsStr_10ms_sys/3(GbISP_TFThmRnwyfDet_flg)
  GbWSM_TplWkUpPrs_flg/1 -> DataFastAbsStr_10ms_sys/4(GbWSM_TplWkUpPrs_flg)
  GbISP_TFHvilLFlt_flg/1 -> DataFastAbsStr_10ms_sys/5(GbISP_TFHvilLFlt_flg)
  GbISP_TFHvilSTG_flg/1 -> DataFastAbsStr_10ms_sys/6(GbISP_TFHvilSTG_flg)
  GbISP_TFHvilSTV_flg/1 -> DataFastAbsStr_10ms_sys/7(GbISP_TFHvilSTV_flg)
  GbISP_TFIsoHVoffResFltLevel1_flg/1 -> DataFastAbsStr_10ms_sys/8(GbISP_TFIsoHVoffResFltLevel1_flg)
  GbISP_TFIsoHVoffResFltLevel2_flg/1 -> DataFastAbsStr_10ms_sys/9(GbISP_TFIsoHVoffResFltLevel2_flg)
  GbISP_TFIsoResFltLevel1_flg/1 -> DataFastAbsStr_10ms_sys/10(GbISP_TFIsoResFltLevel1_flg)
  GbISP_TFIsoResFltLevel2_flg/1 -> DataFastAbsStr_10ms_sys/11(GbISP_TFIsoResFltLevel2_flg)
  GbISP_TFIsoDCResFltLevel1_flg/1 -> DataFastAbsStr_10ms_sys/12(GbISP_TFIsoDCResFltLevel1_flg)
  GbISP_TFIsoDCResFltLevel2_flg/1 -> DataFastAbsStr_10ms_sys/13(GbISP_TFIsoDCResFltLevel2_flg)
  GbISP_TFCANCrashFlt_flg/1 -> DataFastAbsStr_10ms_sys/14(GbISP_TFCANCrashFlt_flg)
  GbISP_TFHWCrashFlt_flg/1 -> DataFastAbsStr_10ms_sys/15(GbISP_TFHWCrashFlt_flg)
  DataFastAbsStr_10ms_sys/1(GcDAS_ThmRnwyWarnCnt_numb) -> GcDAS_ThmRnwyWarnCnt_numb/1
  DataFastAbsStr_10ms_sys/2(GcDAS_ThmRnwyAlarmCnt_numb) -> GcDAS_ThmRnwyAlarmCnt_numb/1
  DataFastAbsStr_10ms_sys/3(GcDAS_ThmRnwyFaultCnt_numb) -> GcDAS_ThmRnwyFaultCnt_numb/1
  DataFastAbsStr_10ms_sys/4(GcDAS_TPLEventWakeCnt_numb) -> GcDAS_TPLEventWakeCnt_numb/1
  DataFastAbsStr_10ms_sys/5(GcDAS_HVILFailCnt_numb) -> GcDAS_HVILFailCnt_numb/1
  DataFastAbsStr_10ms_sys/6(GcDAS_IsoHVOFFChkCnt_numb) -> GcDAS_IsoHVOFFChkCnt_numb/1
  DataFastAbsStr_10ms_sys/7(GcDAS_IsoHVONChkCnt_numb) -> GcDAS_IsoHVONChkCnt_numb/1
  DataFastAbsStr_10ms_sys/8(GcDAS_IsoDCChrgChkCnt_numb) -> GcDAS_IsoDCChrgChkCnt_numb/1
  DataFastAbsStr_10ms_sys/9(GcDAS_CrashNplCnt_numb) -> GcDAS_CrashNplCnt_numb/1
  DataFastAbsStr_10ms_sys/10(GbDAS_HVSafetyNVMStore_flg) -> GbDAS_HVSafetyNVMStore_flg/1
